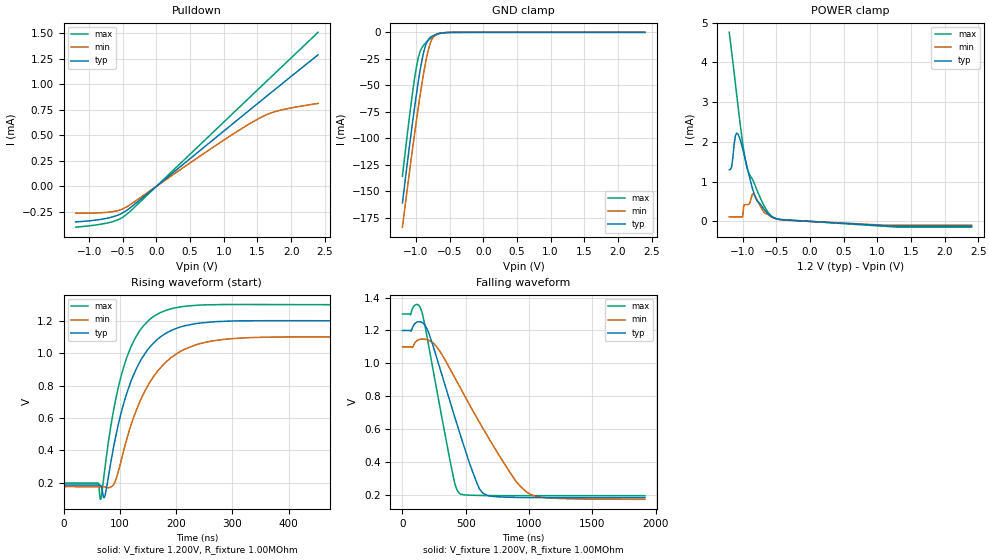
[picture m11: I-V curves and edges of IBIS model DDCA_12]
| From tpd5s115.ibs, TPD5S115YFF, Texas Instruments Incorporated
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[Model]   DDCA_12
Model_type   I/O_open_sink
Vinl = 800.000mV
Vinh = 2.000V
Vmeas = 1.500V
Cref = 15pF
Rref = 1000000
Vref = 0V
|   typ   min   max
|3-state
C_comp   1.2375pF   1.2159pF   1.2825pF
|pulldown
|C_comp   1.2375pF   1.216pF   1.2825pF
[Voltage Range]   1.200V   1.100V   1.300V
|Junction temperature
[Temperature Range]   40.0   100.0   -40.0
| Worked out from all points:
|   slope of the pulldown table from 0 to 0.18 V, typ, clamps not added: 1.84 kohm
|   GND clamp passes 1 mA (typ) near -0.64 V on its own axis
|   POWER clamp passes 1 mA (typ) near -0.88 V on its own axis
|   falling waveform, V_fixture 1.200V, R_fixture 1.00MOhm: 20-80 % time 247ns typ, 419ns min, 160ns max; typ from 1.2 V to 0.185 V
|   rising waveform, V_fixture 1.200V, R_fixture 1.00MOhm: 20-80 % time 57.3ns typ, 69.6ns min, 46.9ns max; typ from 0.185 V to 1.2 V
|ambient temperature   25   85   -40|
[Pulldown]
|   Voltage   I(typ)   I(min)   I(max)
-1.2V     -349uA     -263uA     -400.3uA
-910.6mV  -331.8uA   -261.2uA   -379.7uA
-693.5mV  -307uA     -252.1uA   -353.9uA
-548.7mV  -275.6uA   -233.2uA   -320.6uA
-440.2mV  -234.7uA   -200.8uA   -273.3uA
898.5mV   486.5uA    408uA      565.7uA
1.26V     681.2uA    563uA      793.3uA
1.532V    826.8uA    668.3uA    963.8uA
1.676V    904.2uA    713uA      1.055mA
1.821V    981.4uA    742.6uA    1.146mA
2.4V      1.288mA    812.1uA    1.509mA
[GND Clamp]
|   Voltage   I(typ)   I(min)   I(max)
-1.2V     -160.9mA   -183.7mA   -135.7mA
-1.128V   -123.5mA   -147.5mA   -96.24mA
-1.055V   -87.61mA   -112.4mA   -59.51mA
-1.001V   -62.34mA   -87.12mA   -35.82mA
-964.8mV  -46.72mA   -70.98mA   -23.96mA
-910.6mV  -26.39mA   -48.32mA   -14.55mA
-856.3mV  -12.33mA   -28.52mA   -10.14mA
-820.1mV  -7.344mA   -17.81mA   -7.859mA
-783.9mV  -4.748mA   -9.908mA   -5.874mA
-711.6mV  -2.215mA   -2.556mA   -2.812mA
-476.4mV  -100.5uA   -89.62uA   -87.76uA
2.4V      0A         0A         0A
[POWER Clamp]
|   Voltage   I(typ)   I(min)   I(max)
-1.2V     1.301mA    114.1uA    4.759mA
-1.164V   1.376mA    113.7uA    4.266mA
-1.11V    2.148mA    112.9uA    3.485mA
-1.091V   2.222mA    112.6uA    3.222mA
-1.001V   1.832mA    112uA      1.979mA
-982.9mV  1.709mA    411.5uA    1.769mA
-946.7mV  1.452mA    423.1uA    1.426mA
-856.3mV  837.5uA    689.2uA    1.064mA
-802mV    565.3uA    599.6uA    849.4uA
-675.4mV  290.3uA    215uA      371.3uA
-566.8mV  117.9uA    106uA      127.7uA
2.4V      -117.9uA   -94.86uA   -144.7uA
[Ramp]
R_load = 1.00MOhm
|   typ   min   max
dV/dt_r   609.156mV/57.309ns  554.964mV/69.580ns  661.696mV/46.949ns
dV/dt_f   609.156mV/247.435ns 554.964mV/419.327ns 661.696mV/160.056ns
[Falling Waveform]
V_fixture = 1.200V
V_fixture_min = 1.100V
V_fixture_max = 1.300V
R_fixture = 1.00MOhm
|   Time   V(typ)   V(min)   V(max)
0s        1.2V       1.1V       1.3V
64ns      1.2V       1.1V       1.295V
110ns     1.249V     1.135V     1.357V
150ns     1.25V      1.148V     1.32V
215ns     1.169V     1.138V     1.075V
410ns     681.2mV    917.4mV    281.8mV
454ns     573.5mV    854.7mV    208.4mV
632ns     216mV      610.5mV    198.3mV
995ns     185.7mV    212.2mV    197.2mV
1.914us   184.7mV    175mV      197.2mV
[Rising Waveform]
V_fixture = 1.200V
V_fixture_min = 1.100V
V_fixture_max = 1.300V
R_fixture = 1.00MOhm
|   Time   V(typ)   V(min)   V(max)
0s        184.7mV    175mV      197.2mV
62ns      184.7mV    175mV      196.5mV
66ns      182.2mV    175.1mV    96.67mV
74ns      123.4mV    173.1mV    301.8mV
92ns      473.1mV    208.2mV    702.1mV
117ns     798.9mV    523.3mV    1.015V
155ns     1.045V     829mV      1.214V
208ns     1.163V     1.011V     1.287V
373ns     1.201V     1.1V       1.3V
1.914us   1.2V       1.1V       1.3V
